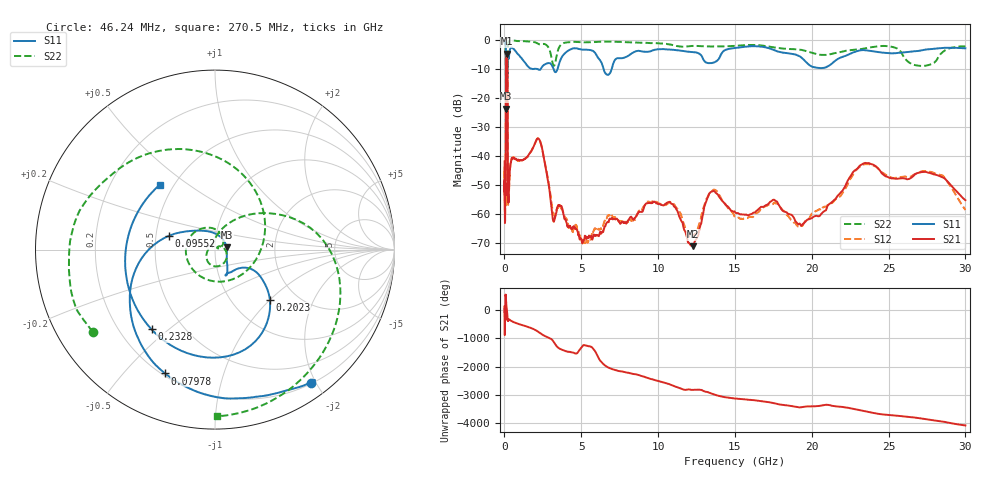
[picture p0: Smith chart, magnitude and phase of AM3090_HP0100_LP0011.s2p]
! Date/Time: Thu, Feb 28, 2019 1:57 PM
! Network Analyzer: Agilent Technologies E8364B Rev: A.07.50.67
! Sweep from 0.010 to 30.000 GHz, 1601 Points, Sweep Type: LOG
! Power Supply: 5.023 V, 0.002 A
# Hz S DB R 50
!freq MagS11 AngS11 MagS21 AngS21 MagS12 AngS12 MagS22 AngS22
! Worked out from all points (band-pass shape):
!   1601 points, 10 MHz to 30 GHz, reference 50 ohm
!   highest |S21| = -4.69 dB at 143.3 MHz (marker M1); lowest = -71.0 dB at 12.25 GHz (marker M2)
!   |S21| within 3 dB of the highest: 104.7 MHz to 188.5 MHz (83.75 MHz wide, 57.1 % of centre)
!   lowest |S11| = -23.7 dB at 103.5 MHz (marker M3), VSWR 1.14, Z = 56.9 + j1.35 ohm
!   |S11| at or under -10 dB: 2.142 GHz to 2.359 GHz (217.5 MHz wide, 9.66 % of centre); 3.195 GHz to 3.455 GHz (259.9 MHz wide, 7.82 % of centre); 6.454 GHz to 6.979 GHz (524.3 MHz wide, 7.81 % of centre)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
!   |S22| runs from -36.8 to -0.2 dB; largest |S21 - S12| = 0.013
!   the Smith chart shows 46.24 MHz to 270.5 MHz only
!   S11 on the Smith chart (normalised r, x): 46.24 MHz: 0.21, -1.94; 79.78 MHz: 0.21, -0.65; 95.52 MHz: 0.59, +0.10; 202.3 MHz: 1.48, -1.00; 232.8 MHz: 0.33, -0.44; 270.5 MHz: 0.42, +0.39
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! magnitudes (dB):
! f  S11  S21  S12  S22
! 10 MHz  -0.3  -41.8  -43.7  -0.6
! 38.04 MHz  -0.5  -60.4  -59.7  -1.4
! 46.24 MHz  -0.8  -51.2  -52.9  -1.7
! 79.78 MHz  -2.6  -48.4  -47.6  -5.2
! 95.52 MHz  -11.5  -15.4  -15.4  -15.2
! 103.5 MHz  -23.7  -8.2  -8.2  -16.4
! 130.3 MHz  -16.3  -4.9  -4.8  -36.8
! 143.3 MHz  -16.5  -4.7  -4.7  -25.0
! 144.7 MHz  -16.5  -4.7  -4.7  -24.1
! 180.3 MHz  -14.3  -6.3  -6.3  -30.4
! 202.3 MHz  -7.7  -15.5  -15.5  -10.6
! 232.8 MHz  -4.9  -55.4  -56.0  -1.5
! 270.5 MHz  -6.5  -55.1  -55.1  -0.6
! 550.5 MHz  -2.9  -40.6  -40.4  -0.2
! 2.084 GHz  -10.0  -34.4  -34.4  -1.0
! 3.204 GHz  -10.1  -62.5  -59.7  -8.9
! 7.926 GHz  -5.8  -62.8  -63.3  -0.8
! 12.25 GHz  -4.2  -71.0  -67.9  -2.0
! 13.61 GHz  -7.8  -52.0  -51.6  -2.2
! 19.41 GHz  -6.4  -63.4  -63.9  -3.5
! 23.59 GHz  -3.6  -42.4  -42.7  -2.8
! 30 GHz  -2.9  -55.2  -58.5  -2.2
